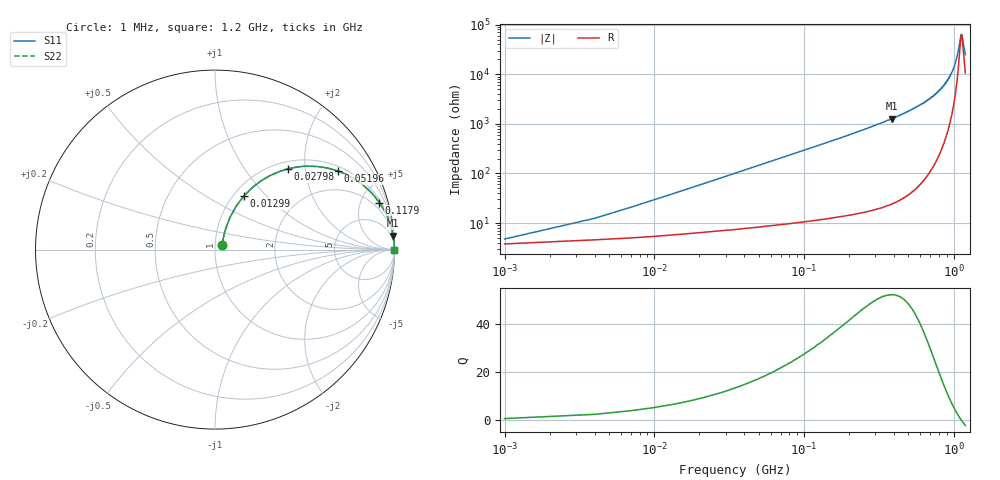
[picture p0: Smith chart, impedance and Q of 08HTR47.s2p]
! Coilcraft 0805HT-R47 Chip Inductor
! 6 August 2004
# MHZ S MA R 50
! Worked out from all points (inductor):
!   401 points, 1 MHz to 1.2 GHz, reference 50 ohm
!   read as one part in series: L = 462 nH near 6.995 MHz
!   highest Q = 52.4 at 387.7 MHz (marker M1), where L = 524 nH
!   self-resonance near 1.128 GHz
!   S11 on the Smith chart (normalised r, x): 1 MHz: 1.08, +0.06; 12.99 MHz: 1.12, +0.75; 27.98 MHz: 1.14, +1.63; 51.96 MHz: 1.17, +3.02; 117.9 MHz: 1.24, +6.92; 1.2 GHz: open
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1  0.046 35.5  0.963 -1.6  0.963 -1.6  0.046 35.5
9.992  0.27 64.0  0.915 -15.4  0.915 -15.4  0.27 64.0
12.99  0.34 61.7  0.891 -19.6  0.891 -19.6  0.34 61.7
18.985  0.463 56.1  0.835 -27.4  0.835 -27.4  0.463 56.1
27.977  0.607 47.9  0.744 -37.2  0.744 -37.2  0.607 47.9
39.968  0.735 39.0  0.631 -47.1  0.631 -47.1  0.735 39.0
51.958  0.814 32.5  0.538 -54.3  0.538 -54.3  0.814 32.5
78.935  0.904 23.1  0.392 -64.5  0.392 -64.5  0.904 23.1
117.903  0.952 16.0  0.275 -72.2  0.275 -72.2  0.952 16.0
201.833  0.983 9.3  0.162 -79.3  0.162 -79.3  0.983 9.3
387.678  0.995 4.5  0.078 -84.4  0.078 -84.4  0.995 4.5
402.665  0.996 4.3  0.074 -84.6  0.074 -84.6  0.996 4.3
600.5  0.998 2.4  0.041 -86.2  0.041 -86.2  0.998 2.4
801.332  0.999 1.2  0.021 -85.9  0.021 -85.9  0.999 1.2
915.237  0.999 0.7  0.013 -83.9  0.013 -83.9  0.999 0.7
1002.165  0.999 0.4  0.007448 -79.2  0.007448 -79.2  0.999 0.4
1056.12  0.999 0.2  0.004367 -70.6  0.004367 -70.6  0.999 0.2
1113.072  0.998 0.1  0.001801 -31.1  0.001801 -31.1  0.998 0.1
1125.062  0.998 0.0  0.001591 -10.1  0.001591 -10.1  0.998 0.0
1143.047  0.998 -0.0  0.001743 23.0  0.001743 23.0  0.998 -0.0
1179.017  0.998 -0.1  0.003067 56.6  0.003067 56.6  0.998 -0.1
1200  0.998 -0.2  0.004027 64.4  0.004027 64.4  0.998 -0.2
